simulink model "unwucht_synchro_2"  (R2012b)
settings: Solver=ode45  StartTime=0.0  StopTime=10.0  RelTol=1e-3
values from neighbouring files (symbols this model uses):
  b = 1    [feder_masse_1.m]    (also in feder_masse_11.m; feder_masse_12.m; unwucht_synchro1.m = 1.25)
  c = 2200    [coulomb_1.m]    (also in coulomb_10.m = 0.1; coulomb_11.m = 0; coulomb_2.m; coulomb_3.m)
  dphi10 = 20    [unwucht_synchro1.m]
  dphi20 = 0    [unwucht_synchro1.m]
  epsilon1 = 0.01    [unwucht_synchro1.m]
  epsilon2 = epsilon1    (= 0.01)    [unwucht_synchro1.m]
  J1 = 1e-5    (= 1e-05)    [unwucht_synchro1.m]
  J2 = J1    (= 1e-05)    [unwucht_synchro1.m]
  k1 = 5000    [feder_masse_1.m]    (also in feder_masse_11.m; feder_masse_13.m; feder_masse_14.m; tilger_gleitreib21.m)
  k2 = mu*k1/((1+mu)^2)    (= 226.757369615)    [feder_masse_1.m]    (also in feder_masse_13.m; feder_masse_14.m; tilger_gleitreib21.m; unwucht_synchro1.m = 5e-05)
  L10 = 25e-4    (= 0.0025)    [unwucht_synchro1.m]
  L20 = 24.5e-4    (= 0.00245)    [unwucht_synchro1.m]
  M = [ms 0;0 ma]    [rad_aufhaeng_1.m]    (also in rad_aufhaeng_2.m; rad_aufhaeng_3.m; rad_aufhaeng_4.m; suspension_1.m = [I 0 0 0;0 ms 0 0;0 0 ma 0;0 0 0 ma])
  m1 = 100    [feder_masse_1.m]    (also in feder_masse_11.m; feder_masse_13.m; feder_masse_14.m; position_reg_2.m = 1)
  m2 = 5    [feder_masse_1.m]    (also in feder_masse_13.m; feder_masse_14.m; foerd_gleit_1.m = 0.1; tilger_gleitreib21.m)
  phi10 = 0    [unwucht_synchro1.m]
  phi20 = 0    [unwucht_synchro1.m]
libraries: simulink x1

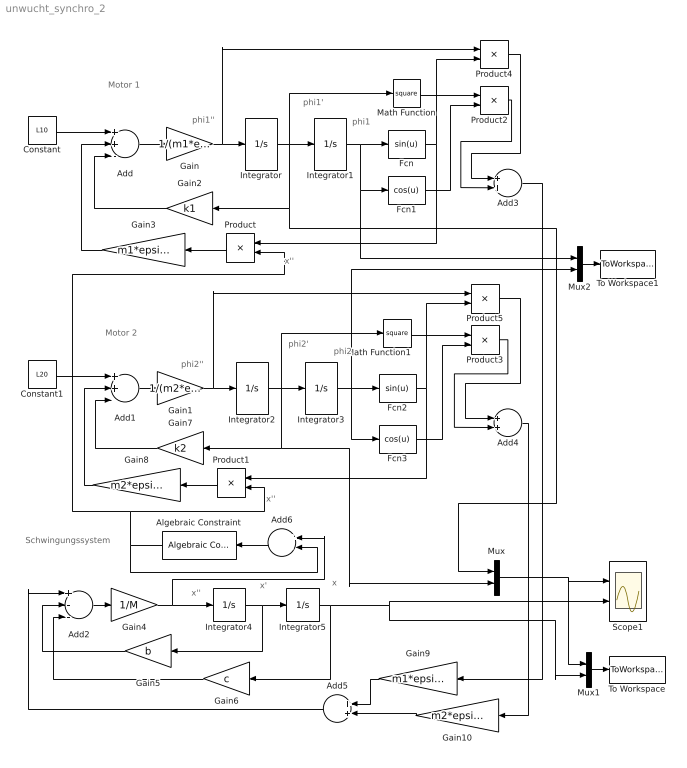
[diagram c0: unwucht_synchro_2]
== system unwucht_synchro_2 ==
  note: x''
  note: x''
  note: Schwingungssystem
  note: Motor 2
  note: Motor 1
  note: phi2
  note: phi2'
  note: phi2''
  note: x
  note: x'
  note: x''
  note: phi1
  note: phi1'
  note: phi1''
  Add : Sum  Inputs=++-
  Add1 : Sum  Inputs=++-
  Add2 : Sum  Inputs=+--
  Add3 : Sum
  Add4 : Sum
  Add5 : Sum
  Add6 : Sum  Inputs=+-
  Algebraic Constraint : simulink/Math Operations/Algebraic Constraint  z0=0
  Constant : Constant  Value=L10
  Constant1 : Constant  Value=L20
  Fcn : Fcn  Expr=sin(u)
  Fcn1 : Fcn  Expr=cos(u)
  Fcn2 : Fcn  Expr=sin(u)
  Fcn3 : Fcn  Expr=cos(u)
  Gain : Gain  Gain=1/(m1*epsilon1^2 + J1)
  Gain1 : Gain  Gain=1/(m2*epsilon2^2 + J2)
  Gain10 : Gain  Gain=m2*epsilon2
  Gain2 : Gain  Gain=k1
  Gain3 : Gain  Gain=m1*epsilon1
  Gain4 : Gain  Gain=1/M
  Gain5 : Gain  Gain=b
  Gain6 : Gain  Gain=c
  Gain7 : Gain  Gain=k2
  Gain8 : Gain  Gain=m2*epsilon2
  Gain9 : Gain  Gain=m1*epsilon1
  Integrator : Integrator  InitialCondition=dphi10
  Integrator1 : Integrator  InitialCondition=phi10
  Integrator2 : Integrator  InitialCondition=phi20
  Integrator3 : Integrator  InitialCondition=dphi20
  Integrator4 : Integrator
  Integrator5 : Integrator
  Math Function : Math  Operator=square
  Math Function1 : Math  Operator=square
  Mux : Mux  Inputs=2
  Mux1 : Mux  Inputs=2
  Mux2 : Mux  Inputs=2
  Product{,1..5} (6 alike) : Product
  Scope1 : Scope  NumInputPorts=2
  To Workspace : ToWorkspace  VariableName=y  SampleTime=-1  SaveFormat=Structure With Time
  To Workspace1 : ToWorkspace  VariableName=phi  SampleTime=-1  SaveFormat=Structure With Time
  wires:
  Constant/1 -> Add/1
  Add/1 -> Gain/1
  Gain/1 -> Product4/1, Integrator/1
  Integrator1/1 -> Fcn1/1, Mux2/1, Fcn/1
  Constant1/1 -> Add1/1
  Add1/1 -> Gain1/1
  Gain1/1 -> Product5/1, Integrator2/1
  Integrator3/1 -> Mux2/2, Fcn2/1, Fcn3/1
  Gain2/1 -> Add/3
  Gain3/1 -> Add/2
  Product/1 -> Gain3/1
  Fcn/1 -> Product/1, Product4/2
  Add5/1 -> Add2/1
  Add2/1 -> Gain4/1
  Gain4/1 -> Add6/1, Integrator4/1
  Integrator4/1 -> Gain5/1, Integrator5/1
  Integrator5/1 -> Gain6/1, Mux1/2, Scope1/2
  Gain5/1 -> Add2/2
  Gain6/1 -> Add2/3
  Gain7/1 -> Add1/3
  Gain8/1 -> Add1/2
  Product1/1 -> Gain8/1
  Fcn2/1 -> Product1/1, Product5/2
  Math Function/1 -> Product2/1
  Fcn1/1 -> Product2/2
  Math Function1/1 -> Product3/1
  Fcn3/1 -> Product3/2
  Product4/1 -> Add3/1
  Product2/1 -> Add3/2
  Product5/1 -> Add4/1
  Product3/1 -> Add4/2
  Add3/1 -> Gain9/1
  Add4/1 -> Gain10/1
  Gain9/1 -> Add5/1
  Gain10/1 -> Add5/2
  Integrator2/1 -> Math Function1/1, Integrator3/1, Mux/2, Gain7/1
  Integrator/1 -> Math Function/1, Mux/1, Gain2/1, Integrator1/1
  Mux/1 -> Mux1/1, Scope1/1
  Mux2/1 -> To Workspace1/1
  Mux1/1 -> To Workspace/1
  Add6/1 -> Algebraic Constraint/1
  Algebraic Constraint/1 -> Add6/2, Product/2, Product1/2
